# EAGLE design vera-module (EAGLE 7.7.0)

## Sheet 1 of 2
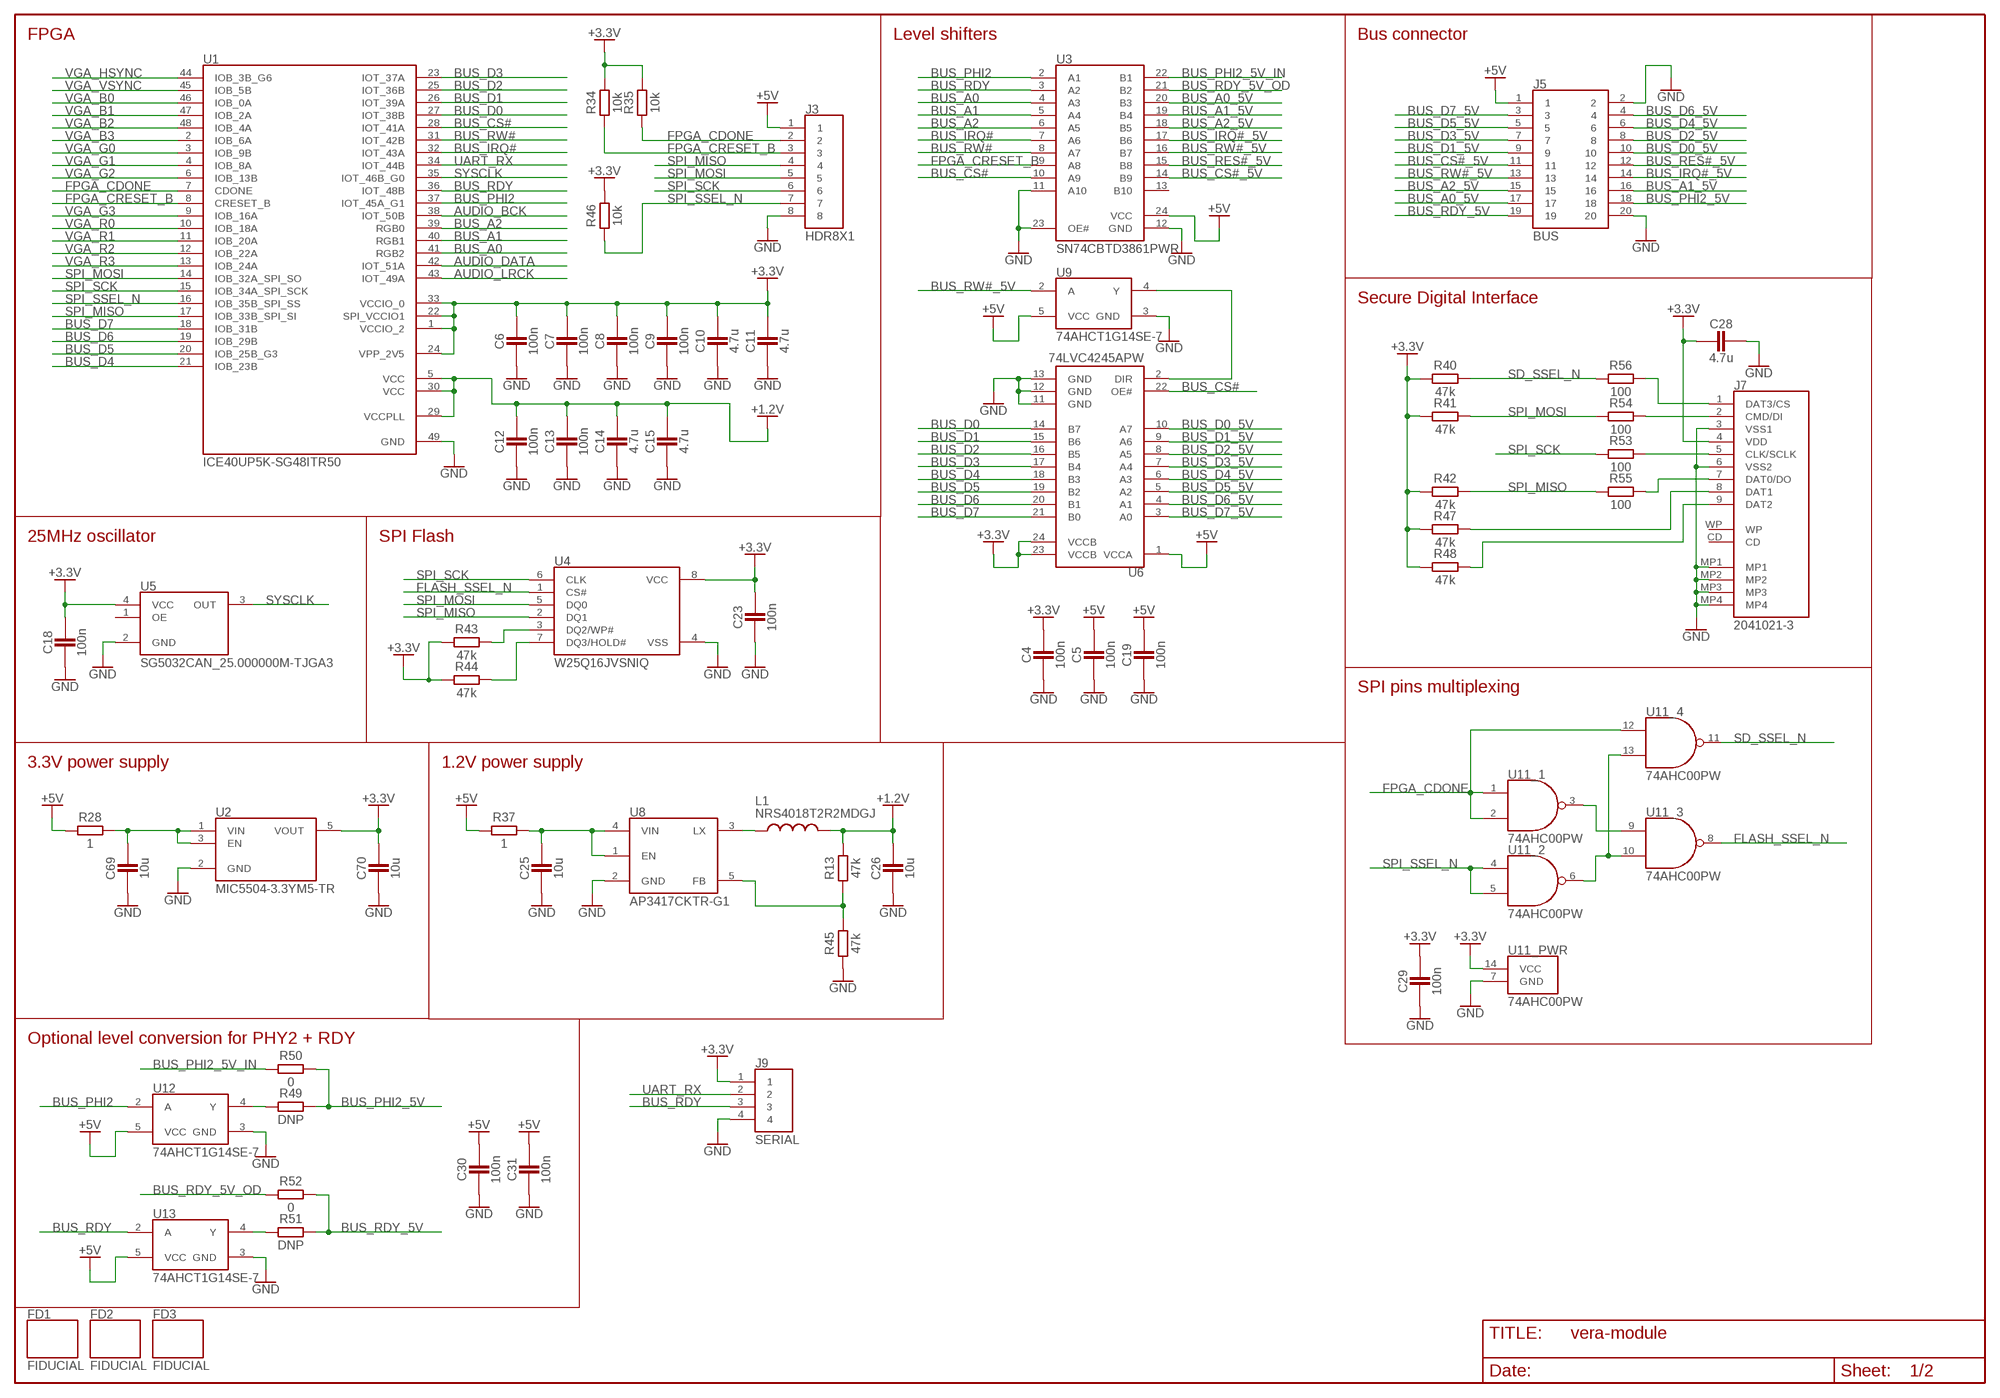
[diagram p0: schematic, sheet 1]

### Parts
C4  100n  CAPACITOR0603  [C0603]
C5  100n  CAPACITOR0603  [C0603]
C6  100n  CAPACITOR0603  [C0603]
C7  100n  CAPACITOR0603  [C0603]
C8  100n  CAPACITOR0603  [C0603]
C9  100n  CAPACITOR0603  [C0603]
C10  4.7u  CAPACITOR0603  [C0603]
C11  4.7u  CAPACITOR0603  [C0603]
C12  100n  CAPACITOR0603  [C0603]
C13  100n  CAPACITOR0603  [C0603]
C14  4.7u  CAPACITOR0603  [C0603]
C15  4.7u  CAPACITOR0603  [C0603]
C18  100n  CAPACITOR0603  [C0603]
C19  100n  CAPACITOR0603  [C0603]
C23  100n  CAPACITOR0603  [C0603]
C25  10u  CAPACITOR0805  [C0805]
C26  10u  CAPACITOR0805  [C0805]
C28  4.7u  CAPACITOR0603  [C0603]
C29  100n  CAPACITOR0603  [C0603]
C30  100n  CAPACITOR0603  [C0603]
C31  100n  CAPACITOR0603  [C0603]
C69  10u  CAPACITOR0805  [C0805]
C70  10u  CAPACITOR0805  [C0805]
FD1  FIDUCIAL  [FIDUCIAL]
FD2  FIDUCIAL  [FIDUCIAL]
FD3  FIDUCIAL  [FIDUCIAL]
J3  HDR8X1  [HDR8X1]
J5  BUS  HDR2X10  [HDR2X10]
J7  2041021-3  [2041021-3]
J9  SERIAL  HDR4X1  [HDR4X1]
L1  NRS4018T2R2MDGJ  INDUCTORNRS4018  [NRS4018]
R13  47k  RESISTOR0603  [R0603]
R28  1  RESISTOR0603  [R0603]
R34  10k  RESISTOR0603  [R0603]
R35  10k  RESISTOR0603  [R0603]
R37  1  RESISTOR0603  [R0603]
R40  47k  RESISTOR0603  [R0603]
R41  47k  RESISTOR0603  [R0603]
R42  47k  RESISTOR0603  [R0603]
R43  47k  RESISTOR0603  [R0603]
R44  47k  RESISTOR0603  [R0603]
R45  47k  RESISTOR0603  [R0603]
R46  10k  RESISTOR0603  [R0603]
R47  47k  RESISTOR0603  [R0603]
R48  47k  RESISTOR0603  [R0603]
R49  DNP  RESISTOR0603  [R0603]
R50  0  RESISTOR0603  [R0603]
R51  DNP  RESISTOR0603  [R0603]
R52  0  RESISTOR0603  [R0603]
R53  100  RESISTOR0603  [R0603]
R54  100  RESISTOR0603  [R0603]
R55  100  RESISTOR0603  [R0603]
R56  100  RESISTOR0603  [R0603]
U1  ICE40UP5K-SG48ITR50  [QFN-48]
U2  MIC5504-3.3YM5-TR  [SOT-23-5]
U3  SN74CBTD3861PWR  [TSSOP-24]
U4  W25Q16JVSNIQ  QSPI_FLASHSOIC8  [SOIC-8]
U5  SG5032CAN_25.000000M-TJGA3  SG5032CAN_40.000000M-TJGA3  [SG5032]
U6  74LVC4245APW  [TSSOP-24]
U8  AP3417CKTR-G1  [SOT-23-5]
U9  74AHCT1G14SE-7  [TSSOP-5]
U11  74AHC00PW  [TSSOP-14]
U12  74AHCT1G14SE-7  [TSSOP-5]
U13  74AHCT1G14SE-7  [TSSOP-5]

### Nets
+1.2V: C12.2 C13.2 C14.2 C15.2 C26.2 L1.2 R13.2 U1.5(VCC) U1.29(VCCPLL) U1.30(VCC)
+3.3V: C4.2 C6.2 C7.2 C8.2 C9.2 C10.2 C11.2 C18.2 C23.2 C28.1 C29.2 C70.2 J7.4(VDD) J9.1 R34.1 R35.1 R40.1 R41.1 R42.1 R43.1 R44.1 R46.1 R47.1 R48.1 U1.1(VCCIO_2) U1.22(SPI_VCCIO1) U1.24(VPP_2V5) U1.33(VCCIO_0) U2.5(VOUT) U4.8(VCC) U5.4(VCC) U6.23(VCCB) U6.24(VCCB) U11.14(_PWR:VCC) ; also sheet 2
+5V [5V]: C5.2 C19.2 C30.2 C31.2 J3.1 J5.1 R28.1 R37.1 U3.24(VCC) U6.1(VCCA) U9.5(VCC) U12.5(VCC) U13.5(VCC)
AUDIO_BCK: U1.38(IOT_50B) ; also sheet 2
AUDIO_DATA: U1.42(IOT_51A) ; also sheet 2
AUDIO_LRCK: U1.43(IOT_49A) ; also sheet 2
BUS_A0: U1.41(RGB2) U3.4(A3)
BUS_A0_5V: J5.17 U3.20(B3)
BUS_A1: U1.40(RGB1) U3.5(A4)
BUS_A1_5V: J5.16 U3.19(B4)
BUS_A2: U1.39(RGB0) U3.6(A5)
BUS_A2_5V: J5.15 U3.18(B5)
BUS_CS#: U1.28(IOT_41A) U3.10(A9) U6.22(OE#)
BUS_CS#_5V: J5.11 U3.14(B9)
BUS_D0: U1.27(IOT_38B) U6.14(B7)
BUS_D0_5V: J5.10 U6.10(A7)
BUS_D1: U1.26(IOT_39A) U6.15(B6)
BUS_D1_5V: J5.9 U6.9(A6)
BUS_D2: U1.25(IOT_36B) U6.16(B5)
BUS_D2_5V: J5.8 U6.8(A5)
BUS_D3: U1.23(IOT_37A) U6.17(B4)
BUS_D3_5V: J5.7 U6.7(A4)
BUS_D4: U1.21(IOB_23B) U6.18(B3)
BUS_D4_5V: J5.6 U6.6(A3)
BUS_D5: U1.20(IOB_25B_G3) U6.19(B2)
BUS_D5_5V: J5.5 U6.5(A2)
BUS_D6: U1.19(IOB_29B) U6.20(B1)
BUS_D6_5V: J5.4 U6.4(A1)
BUS_D7: U1.18(IOB_31B) U6.21(B0)
BUS_D7_5V: J5.3 U6.3(A0)
BUS_IRQ#: U1.32(IOT_43A) U3.7(A6)
BUS_IRQ#_5V: J5.14 U3.17(B6)
BUS_PHI2: U1.37(IOT_45A_G1) U3.2(A1) U12.2(A)
BUS_PHI2_5V: J5.18 R49.2 R50.2
BUS_PHI2_5V_IN: R50.1 U3.22(B1)
BUS_RDY: J9.3 U1.36(IOT_48B) U3.3(A2) U13.2(A)
BUS_RDY_5V: J5.19 R51.2 R52.2
BUS_RDY_5V_OD: R52.1 U3.21(B2)
BUS_RES#_5V: J5.12 U3.15(B8)
BUS_RW#: U1.31(IOT_42B) U3.8(A7)
BUS_RW#_5V: J5.13 U3.16(B7) U9.2(A)
FLASH_SSEL_N: U4.1(CS#) U11.8(_3:Y)
FPGA_CDONE: J3.2 R35.2 U1.7(CDONE) U11.1(_1:A) U11.2(_1:B) U11.12(_4:A)
FPGA_CRESET_B: J3.3 R34.2 U1.8(CRESET_B) U3.9(A8)
GND: C4.1 C5.1 C6.1 C7.1 C8.1 C9.1 C10.1 C11.1 C12.1 C13.1 C14.1 C15.1 C18.1 C19.1 C23.1 C25.1 C26.1 C28.2 C29.1 C30.1 C31.1 C69.1 C70.1 J3.8 J5.2 J5.20 J7.3(VSS1) J7.6(VSS2) J7.MP1 J7.MP2 J7.MP3 J7.MP4 J9.4 R45.1 U1.49(GND) U2.2(GND) U3.11(A10) U3.12(GND) U3.23(OE#) U4.4(VSS) U5.2(GND) U6.11(GND) U6.12(GND) U6.13(GND) U8.2(GND) U9.3(GND) U11.7(_PWR:GND) U12.3(GND) U13.3(GND) ; also sheet 2
N$7: C69.2 R28.2 U2.1(VIN) U2.3(EN)
N$8: U6.2(DIR) U9.4(Y)
N$14: R43.2 U4.3(DQ2/WP#)
N$15: R13.1 R45.2 U8.5(FB)
N$19: R44.2 U4.7(DQ3/HOLD#)
N$20: L1.1 U8.3(LX)
N$22 [5V]: C25.2 R37.2 U8.1(EN) U8.4(VIN)
N$43: J7.8(DAT1) R47.2
N$44: J7.9(DAT2) R48.2
N$46: U11.3(_1:Y) U11.9(_3:A)
N$47: U11.6(_2:Y) U11.10(_3:B) U11.13(_4:B)
N$48: R49.1 U12.4(Y)
N$50: R51.1 U13.4(Y)
N$51: J7.2(CMD/DI) R54.2
N$52: J7.5(CLK/SCLK) R53.2
N$53: J7.1(DAT3/CS) R56.2
N$54: J7.7(DAT0/DO) R55.2
SD_SSEL_N: R40.2 R56.1 U11.11(_4:Y)
SPI_MISO: J3.4 R42.2 R55.1 U1.17(IOB_33B_SPI_SI) U4.2(DQ1)
SPI_MOSI: J3.5 R41.2 R54.1 U1.14(IOB_32A_SPI_SO) U4.5(DQ0)
SPI_SCK: J3.6 R53.1 U1.15(IOB_34A_SPI_SCK) U4.6(CLK)
SPI_SSEL_N: J3.7 R46.2 U1.16(IOB_35B_SPI_SS) U11.4(_2:A) U11.5(_2:B)
SYSCLK: U1.35(IOT_46B_G0) U5.3(OUT) ; also sheet 2
UART_RX: J9.2 U1.34(IOT_44B)
VGA_B0: U1.46(IOB_0A) ; also sheet 2
VGA_B1: U1.47(IOB_2A) ; also sheet 2
VGA_B2: U1.48(IOB_4A) ; also sheet 2
VGA_B3: U1.2(IOB_6A) ; also sheet 2
VGA_G0: U1.3(IOB_9B) ; also sheet 2
VGA_G1: U1.4(IOB_8A) ; also sheet 2
VGA_G2: U1.6(IOB_13B) ; also sheet 2
VGA_G3: U1.9(IOB_16A) ; also sheet 2
VGA_HSYNC: U1.44(IOB_3B_G6) ; also sheet 2
VGA_R0: U1.10(IOB_18A) ; also sheet 2
VGA_R1: U1.11(IOB_20A) ; also sheet 2
VGA_R2: U1.12(IOB_22A) ; also sheet 2
VGA_R3: U1.13(IOB_24A) ; also sheet 2
VGA_VSYNC: U1.45(IOB_5B) ; also sheet 2
Unconnected: J7.CD J7.WP U3.13(B10) U5.1(OE)

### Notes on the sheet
- FPGA | Level shifters | Bus connector
- Secure Digital Interface
- 25MHz oscillator | SPI Flash
- SPI pins multiplexing
- 3.3V power supply | 1.2V power supply
- Optional level conversion for PHY2 + RDY

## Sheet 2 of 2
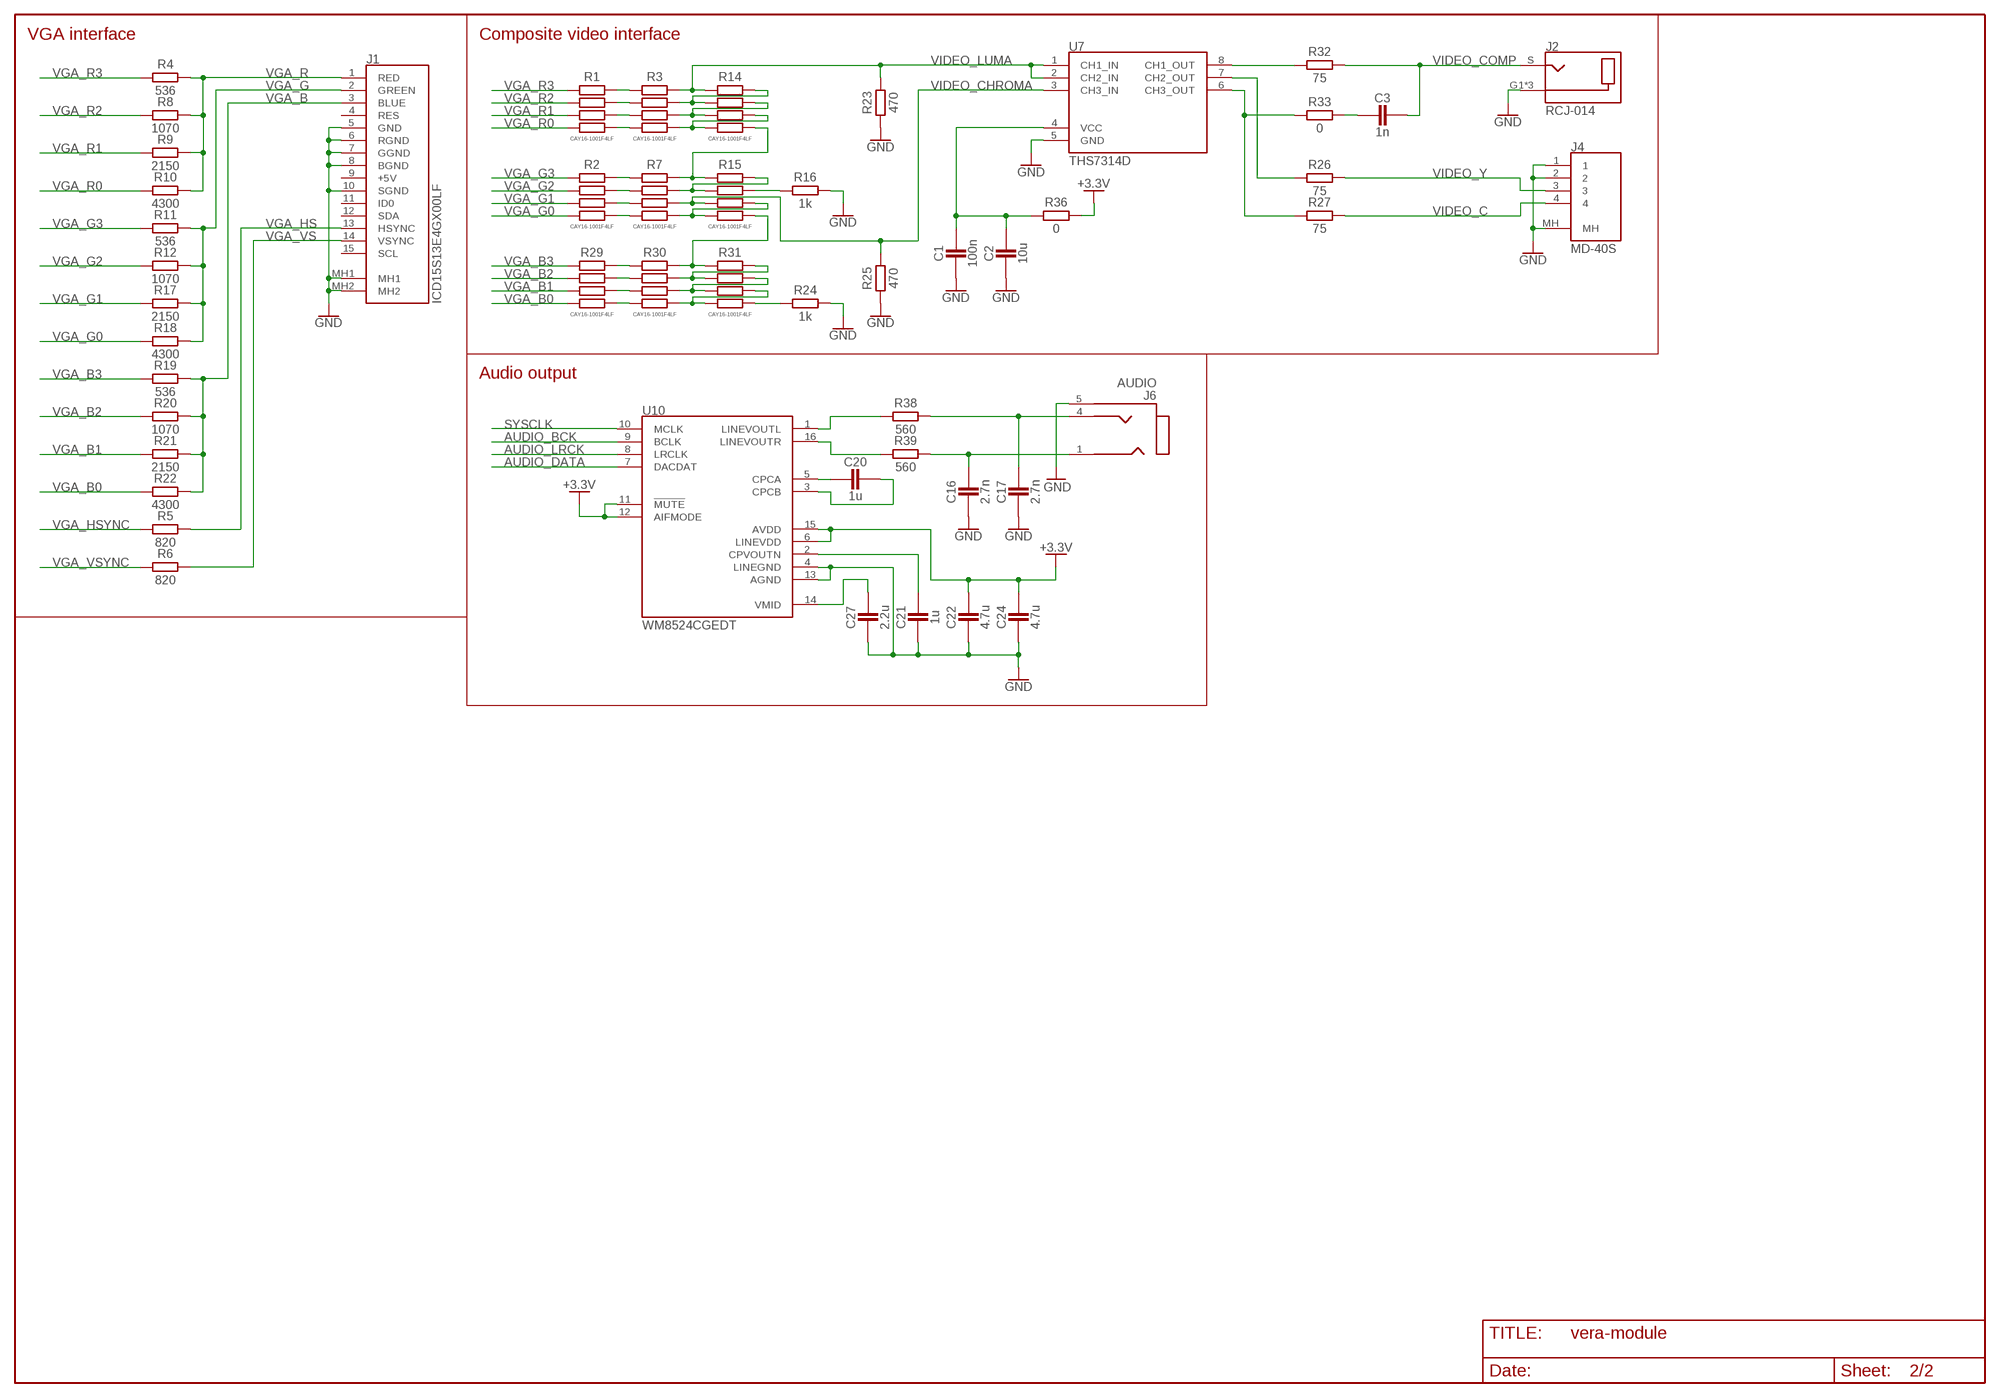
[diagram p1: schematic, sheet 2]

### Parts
C1  100n  CAPACITOR0603  [C0603]
C2  10u  CAPACITOR0805  [C0805]
C3  1n  CAPACITOR0603  [C0603]
C16  2.7n  CAPACITOR0603  [C0603]
C17  2.7n  CAPACITOR0603  [C0603]
C20  1u  CAPACITOR0603  [C0603]
C21  1u  CAPACITOR0603  [C0603]
C22  4.7u  CAPACITOR0603  [C0603]
C24  4.7u  CAPACITOR0603  [C0603]
C27  2.2u  CAPACITOR0603  [C0603]
J1  ICD15S13E4GX00LF  [1-1734344-2]
J2  RCJ-014  [RCJ-01X]
J4  MD-40S  [MD-40S]
J6  AUDIO  35RASMT2BHNTRX  [35RASMT2BHNTRX]
R1  CAY16-1001F4LF  RES_ARRAY41206  [RA4_1206]
R2  CAY16-1001F4LF  RES_ARRAY41206  [RA4_1206]
R3  CAY16-1001F4LF  RES_ARRAY41206  [RA4_1206]
R4  536  RESISTOR0603  [R0603]
R5  820  RESISTOR0603  [R0603]
R6  820  RESISTOR0603  [R0603]
R7  CAY16-1001F4LF  RES_ARRAY41206  [RA4_1206]
R8  1070  RESISTOR0603  [R0603]
R9  2150  RESISTOR0603  [R0603]
R10  4300  RESISTOR0603  [R0603]
R11  536  RESISTOR0603  [R0603]
R12  1070  RESISTOR0603  [R0603]
R14  CAY16-1001F4LF  RES_ARRAY41206  [RA4_1206]
R15  CAY16-1001F4LF  RES_ARRAY41206  [RA4_1206]
R16  1k  RESISTOR0603  [R0603]
R17  2150  RESISTOR0603  [R0603]
R18  4300  RESISTOR0603  [R0603]
R19  536  RESISTOR0603  [R0603]
R20  1070  RESISTOR0603  [R0603]
R21  2150  RESISTOR0603  [R0603]
R22  4300  RESISTOR0603  [R0603]
R23  470  RESISTOR0603  [R0603]
R24  1k  RESISTOR0603  [R0603]
R25  470  RESISTOR0603  [R0603]
R26  75  RESISTOR0603  [R0603]
R27  75  RESISTOR0603  [R0603]
R29  CAY16-1001F4LF  RES_ARRAY41206  [RA4_1206]
R30  CAY16-1001F4LF  RES_ARRAY41206  [RA4_1206]
R31  CAY16-1001F4LF  RES_ARRAY41206  [RA4_1206]
R32  75  RESISTOR0603  [R0603]
R33  0  RESISTOR0603  [R0603]
R36  0  RESISTOR0603  [R0603]
R38  560  RESISTOR0603  [R0603]
R39  560  RESISTOR0603  [R0603]
U7  THS7314D  [SOIC-8]
U10  WM8524CGEDT  [TSSOP-16]

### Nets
+3.3V: C22.2 C24.2 R36.2 U10.6(LINEVDD) U10.11(!MUTE) U10.12(AIFMODE) U10.15(AVDD) ; also sheet 1
AUDIO_BCK: U10.9(BCLK) ; also sheet 1
AUDIO_DATA: U10.7(DACDAT) ; also sheet 1
AUDIO_LRCK: U10.8(LRCLK) ; also sheet 1
GND: C1.1 C2.1 C16.1 C17.1 C21.1 C22.1 C24.1 C27.1 J1.5(GND) J1.6(RGND) J1.7(GGND) J1.8(BGND) J1.10(SGND) J1.MH1 J1.MH2 J2.G1(G) J2.G2(G) J2.G3(G) J4.1 J4.2 J4.MH J6.5(SLEEVE) R16.2 R23.1 R24.2 R25.1 U7.5(GND) U10.4(LINEGND) U10.13(AGND) ; also sheet 1
N$1: R1.1A R3.1B
N$2: R1.2A R3.2B
N$3: R1.3A R3.3B
N$4: R1.4A R3.4B
N$5: R2.1A R7.1B
N$6: R2.2A R7.2B
N$9: R29.1A R30.1B
N$10: R2.3A R7.3B
N$11: R2.4A R7.4B
N$12: R27.1 R33.1 U7.6(CH3_OUT)
N$13: R3.2A R14.1A R14.2B
N$16: R3.3A R14.2A R14.3B
N$17: R3.4A R14.3A R14.4B
N$18: R7.1A R14.4A R15.1B
N$21: R7.2A R15.1A R15.2B
N$23: R32.1 U7.8(CH1_OUT)
N$24: C3.1 R33.2
N$25: R7.4A R15.3A R15.4B
N$26: C20.2 U10.3(CPCB)
N$27: R29.2A R30.2B
N$28: R29.3A R30.3B
N$29: R15.2A R16.1
N$30: R29.4A R30.4B
N$31: R15.4A R30.1A R31.1B
N$32: R30.2A R31.1A R31.2B
N$33: R30.3A R31.2A R31.3B
N$34: R24.1 R31.4A
N$35: R30.4A R31.3A R31.4B
N$36: R26.1 U7.7(CH2_OUT)
N$37: C1.2 C2.2 R36.1 U7.4(VCC)
N$38: C17.2 J6.4(TIP) R38.2
N$39: C16.2 J6.1(RING) R39.2
N$40: R38.1 U10.1(LINEVOUTL)
N$41: R39.1 U10.16(LINEVOUTR)
N$42: C20.1 U10.5(CPCA)
N$45: C21.2 U10.2(CPVOUTN)
N$49: C27.2 U10.14(VMID)
SYSCLK: U10.10(MCLK) ; also sheet 1
VGA_B: J1.3(BLUE) R19.2 R20.2 R21.2 R22.2
VGA_B0: R22.1 R29.4B ; also sheet 1
VGA_B1: R21.1 R29.3B ; also sheet 1
VGA_B2: R20.1 R29.2B ; also sheet 1
VGA_B3: R19.1 R29.1B ; also sheet 1
VGA_G: J1.2(GREEN) R11.2 R12.2 R17.2 R18.2
VGA_G0: R2.4B R18.1 ; also sheet 1
VGA_G1: R2.3B R17.1 ; also sheet 1
VGA_G2: R2.2B R12.1 ; also sheet 1
VGA_G3: R2.1B R11.1 ; also sheet 1
VGA_HS: J1.13(HSYNC) R5.2
VGA_HSYNC: R5.1 ; also sheet 1
VGA_R: J1.1(RED) R4.2 R8.2 R9.2 R10.2
VGA_R0: R1.4B R10.1 ; also sheet 1
VGA_R1: R1.3B R9.1 ; also sheet 1
VGA_R2: R1.2B R8.1 ; also sheet 1
VGA_R3: R1.1B R4.1 ; also sheet 1
VGA_VS: J1.14(VSYNC) R6.2
VGA_VSYNC: R6.1 ; also sheet 1
VIDEO_C: J4.4 R27.2
VIDEO_CHROMA: R7.3A R15.3B R25.2 U7.3(CH3_IN)
VIDEO_COMP: C3.2 J2.S R32.2
VIDEO_LUMA: R3.1A R14.1B R23.2 U7.1(CH1_IN) U7.2(CH2_IN)
VIDEO_Y: J4.3 R26.2
Unconnected: J1.4(RES) J1.9(+5V) J1.11(ID0) J1.12(SDA) J1.15(SCL)

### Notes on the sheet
- VGA interface | Composite video interface
- Audio output

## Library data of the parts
C1-C31 C69 C70 = rcl:CAPACITOR
FD1-FD3 = misc:FIDUCIAL
J1 = connectors:ICD15S13E4GX00LF
J2 = connectors:RCJ-014
J3 = connectors:HDR8X1
J4 = connectors:MD-40S
J5 = connectors:HDR2X10
J6 = connectors:35RASMT2BHNTRX
J7 = connectors:2041021-3
J9 = connectors:HDR4X1
L1 = rcl:INDUCTOR
R1-R3 R7 R14 R15 R29-R31 = rcl:RES_ARRAY4
R4-R6 R8-R13 R16-R28 R32-R56 = rcl:RESISTOR
U1 = integrated_circuits:ICE40UP5K-SG48ITR50: Lattice ICE40 5K LE FPGA
U2 = integrated_circuits:MIC5504-3.3YM5-TR
U3 = integrated_circuits:SN74CBTD3861PWR
U4 = integrated_circuits:QSPI_FLASH
U5 = integrated_circuits:SG5032CAN_40.000000M-TJGA3: Epson 40 MHz 3.3V Oscillator +/- 50ppm
U6 = integrated_circuits:74LVC4245APW
U7 = integrated_circuits:THS7314D
U8 = integrated_circuits:AP3417CKTR-G1
U9 U12 U13 = integrated_circuits:74AHCT1G14SE-7
U10 = integrated_circuits:WM8524CGEDT
U11 = integrated_circuits:74AHC00PW

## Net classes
1 5V: clearance 0.2 mm

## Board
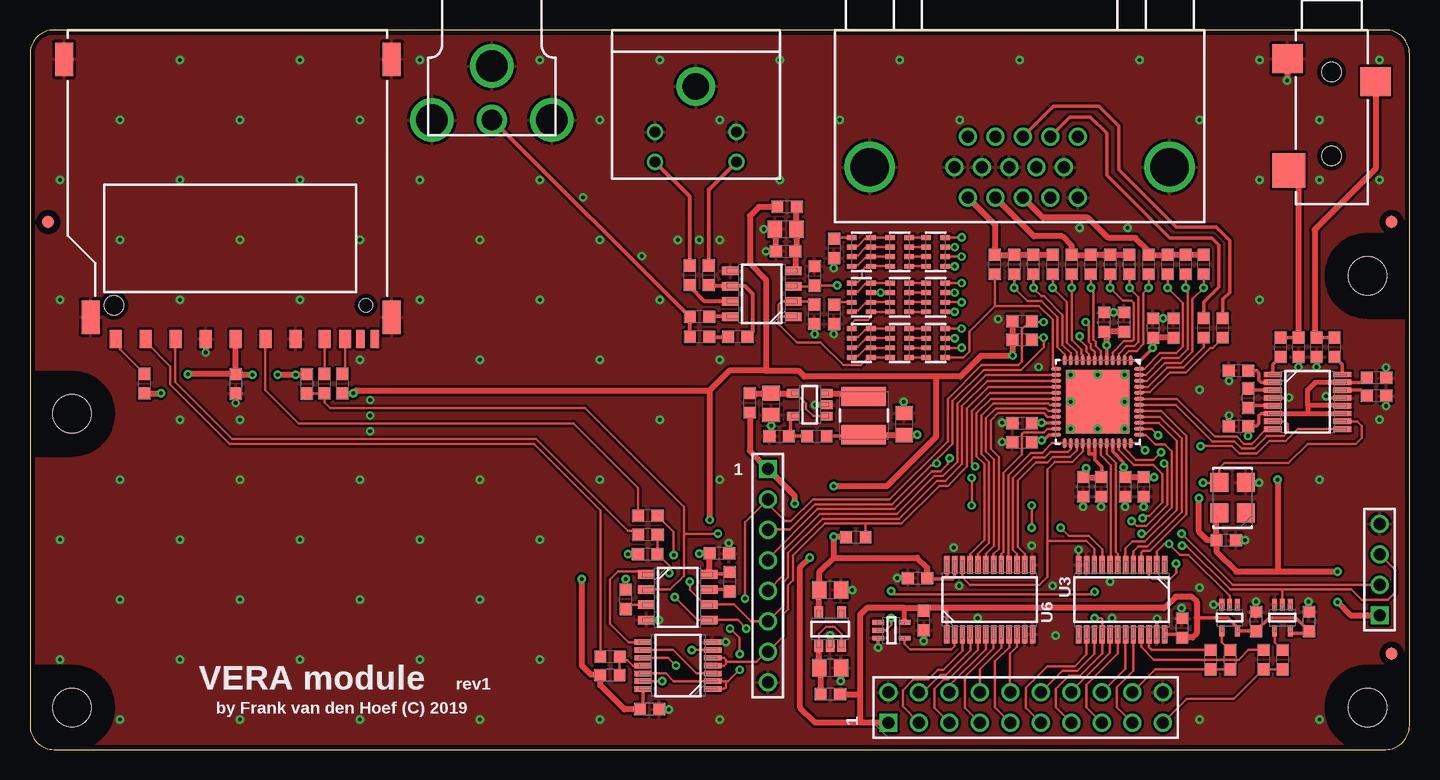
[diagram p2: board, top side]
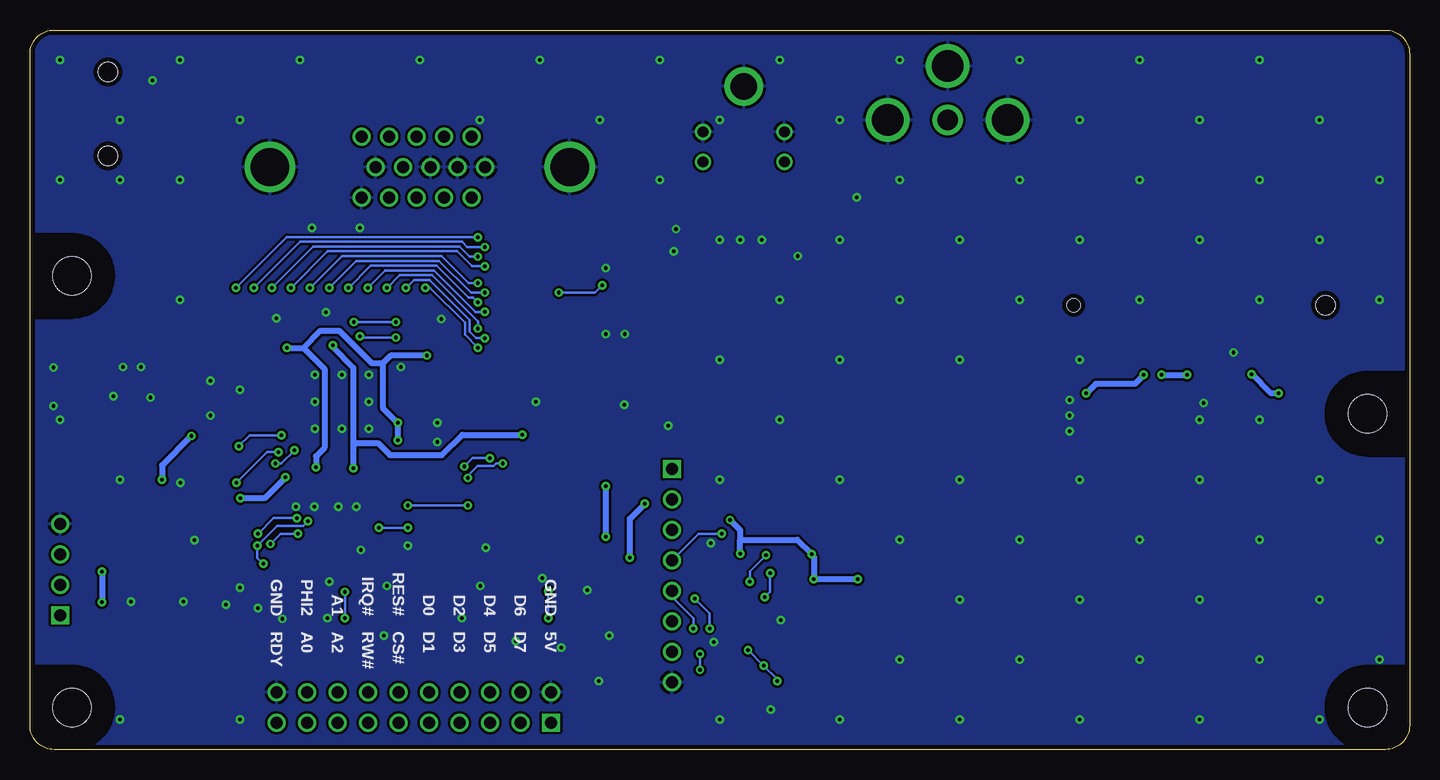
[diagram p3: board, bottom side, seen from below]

Size 115 x 60 mm. Coordinates in mm from the lower left corner, seen from the top.
Outline: 115,2 115,58 arc90 113,60 2,60 arc90 0,58 0,2 arc90 2,0 113,0 arc90 115,2
Copper layers (1*16): Top 0.035mm / dielectric 1.6mm / Bottom 0.035mm
Design rules "Frank_2-layer *": minimum track width 0.2mm, minimum drill 0.3mm, track to track 0.2mm, track to pad 0.2mm, pad to pad 0.2mm, via to via 0.2mm, smd to smd 0mil, copper to edge 0.4mm, drill to drill 10mil, minimum pad ring 0.2mm, minimum via ring 0.2mm, stop-mask expansion 0.1mm, vias tented up to drill 20mil, thermal gap 10mil
Holes 3.2 mm at 3.5,28 3.5,3.5 111.5,3.5 111.5,39.5
tRestrict: area 86,26 to 92,32; area 0,24.5 to 7,31.5; area 0,0 to 7,7; area 108,0 to 115,7; area 108,36 to 115,43
bRestrict: area 0,24.5 to 7,31.5; area 0,0 to 7,7; area 108,0 to 115,7; area 108,36 to 115,43

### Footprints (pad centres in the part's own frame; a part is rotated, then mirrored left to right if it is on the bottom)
C0603 = smd 0.95 x 1: 1 -0.8,0; 2 0.8,0
C0805 = smd 1.15 x 1.45: 1 -0.9,0; 2 0.9,0
FIDUCIAL = smd 1 x 1: FD 0,0
1-1734344-2 = drill 1: 1 4.315,13.97; 2 2.025,13.97; 3 -0.265,13.97; 4 -2.555,13.97; 5 -4.845,13.97; 6 5.455,11.43; 7 3.165,11.43; 8 0.875,11.43; 9 -1.415,11.43; 10 -3.705,11.43; 11 4.315,8.89; 12 2.025,8.89; 13 -0.265,8.89; 14 -2.555,8.89; 15 -4.845,8.89 | drill 3.18: MH1 -12.495,11.43; MH2 12.495,11.43
RCJ-01X = drill 2.6: G1 0,0; G2 -5,-4.5; G3 5,-4.5 | drill 1.7: S 0,-4.5
HDR8X1 = drill 1 square: 1 0,8.89 | drill 1: 2 0,6.35; 3 0,3.81; 4 0,1.27; 5 0,-1.27; 6 0,-3.81; 7 0,-6.35; 8 0,-8.89
MD-40S = drill 0.9: 1 -3.4,-8.5; 2 3.4,-8.5; 3 -3.4,-11; 4 3.4,-11 | drill 2.2: MH 0,-4.7
HDR2X10 = drill 1 square: 1 -1.27,11.43 | drill 1: 2 1.27,11.43; 3 -1.27,8.89; 4 1.27,8.89; 5 -1.27,6.35; 6 1.27,6.35; 7 -1.27,3.81; 8 1.27,3.81; 9 -1.27,1.27; 10 1.27,1.27; 11 -1.27,-1.27; 12 1.27,-1.27; 13 -1.27,-3.81; 14 1.27,-3.81; 15 -1.27,-6.35; 16 1.27,-6.35; 17 -1.27,-8.89; 18 1.27,-8.89; 19 -1.27,-11.43; 20 1.27,-11.43
35RASMT2BHNTRX = smd 2.4 x 2.55: 1 4.3,3.675; 5 2.4,-3.675 | smd 2.9 x 2.75: 4 11.7,-3.575 | hole 1.6: 3.5,0; 10.5,0
2041021-3 = smd 1 x 1.5: 1 6.875,25.75; 2 4.375,25.75; 3 1.875,25.75; 4 -0.625,25.75; 5 -3.125,25.75; 6 -5.625,25.75; 7 -8.055,25.75; 8 -9.755,25.75; 9 9.375,25.75 | smd 0.7 x 1.5: CD -11.055,25.75; WP -12.255,25.75 | smd 1.5 x 2.8: MP1 -13.65,23.95; MP2 11.45,23.95; MP3 -13.65,2.45; MP4 13.65,2.45 | hole 1.1: -11.5,22.95 | hole 1.6: 9.5,22.95
HDR4X1 = drill 1 square: 1 0,3.81 | drill 1: 2 0,1.27; 3 0,-1.27; 4 0,-3.81
NRS4018 = smd 1.6 x 3.7: 1 -1.6,0; 2 1.6,0
RA4_1206 = smd 0.4 x 0.8: 1A -1.2,0.8; 1B -1.2,-0.8; 2A -0.4,0.8; 2B -0.4,-0.8; 3A 0.4,0.8; 3B 0.4,-0.8; 4A 1.2,0.8; 4B 1.2,-0.8
R0603 = smd 0.95 x 1: 1 -0.8,0; 2 0.8,0
QFN-48 = smd 0.85 x 0.3: 1 -3.45,2.75; 2 -3.45,2.25; 3 -3.45,1.75; 4 -3.45,1.25; 5 -3.45,0.75; 6 -3.45,0.25; 7 -3.45,-0.25; 8 -3.45,-0.75; 9 -3.45,-1.25; 10 -3.45,-1.75; 11 -3.45,-2.25; 12 -3.45,-2.75; 25 3.45,-2.75; 26 3.45,-2.25; 27 3.45,-1.75; 28 3.45,-1.25; 29 3.45,-0.75; 30 3.45,-0.25; 31 3.45,0.25; 32 3.45,0.75; 33 3.45,1.25; 34 3.45,1.75; 35 3.45,2.25; 36 3.45,2.75 | smd 0.3 x 0.85: 13 -2.75,-3.45; 14 -2.25,-3.45; 15 -1.75,-3.45; 16 -1.25,-3.45; 17 -0.75,-3.45; 18 -0.25,-3.45; 19 0.25,-3.45; 20 0.75,-3.45; 21 1.25,-3.45; 22 1.75,-3.45; 23 2.25,-3.45; 24 2.75,-3.45; 37 2.75,3.45; 38 2.25,3.45; 39 1.75,3.45; 40 1.25,3.45; 41 0.75,3.45; 42 0.25,3.45; 43 -0.25,3.45; 44 -0.75,3.45; 45 -1.25,3.45; 46 -1.75,3.45; 47 -2.25,3.45; 48 -2.75,3.45 | smd 5.3 x 5.3: 49 0,0
SOT-23-5 = smd 1 x 0.71: 1 -1.4,0.95; 2 -1.4,0; 3 -1.4,-0.95; 4 1.4,-0.95; 5 1.4,0.95
TSSOP-24 = smd 1.5 x 0.45: 1 -2.9,3.575; 2 -2.9,2.925; 3 -2.9,2.275; 4 -2.9,1.625; 5 -2.9,0.975; 6 -2.9,0.325; 7 -2.9,-0.325; 8 -2.9,-0.975; 9 -2.9,-1.625; 10 -2.9,-2.275; 11 -2.9,-2.925; 12 -2.9,-3.575; 13 2.9,-3.575; 14 2.9,-2.925; 15 2.9,-2.275; 16 2.9,-1.625; 17 2.9,-0.975; 18 2.9,-0.325; 19 2.9,0.325; 20 2.9,0.975; 21 2.9,1.625; 22 2.9,2.275; 23 2.9,2.925; 24 2.9,3.575
SOIC-8 = smd 1.35 x 0.71: 1 -2.625,1.905; 2 -2.625,0.635; 3 -2.625,-0.635; 4 -2.625,-1.905; 5 2.625,-1.905; 6 2.625,-0.635; 7 2.625,0.635; 8 2.625,1.905
SG5032 = smd 1.6 x 1.5: 1 -1.27,-1.1; 2 1.27,-1.1; 3 1.27,1.1; 4 -1.27,1.1
TSSOP-5 = smd 0.95 x 0.4: 1 -1.1,0.65; 2 -1.1,0; 3 -1.1,-0.65; 4 1.1,-0.65; 5 1.1,0.65
TSSOP-16 = smd 1.5 x 0.45: 1 -2.9,2.275; 2 -2.9,1.625; 3 -2.9,0.975; 4 -2.9,0.325; 5 -2.9,-0.325; 6 -2.9,-0.975; 7 -2.9,-1.625; 8 -2.9,-2.275; 9 2.9,-2.275; 10 2.9,-1.625; 11 2.9,-0.975; 12 2.9,-0.325; 13 2.9,0.325; 14 2.9,0.975; 15 2.9,1.625; 16 2.9,2.275
TSSOP-14 = smd 1.45 x 0.45: 1 -2.9,1.95; 2 -2.9,1.3; 3 -2.9,0.65; 4 -2.9,0; 5 -2.9,-0.65; 6 -2.9,-1.3; 7 -2.9,-1.95; 8 2.9,-1.95; 9 2.9,-1.3; 10 2.9,-0.65; 11 2.9,0; 12 2.9,0.65; 13 2.9,1.3; 14 2.9,1.95

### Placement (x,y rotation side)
C1  63,41.55 0 top
C2  63,43.4 0 top
C3  55.8,34.4 180 top
C4  74,14.3 0 top
C5  96,10.15 270 top
C6  93.6,35.15 270 top
C7  82.7,27.25 0 top
C8  82.7,25.65 0 top
C9  91.3,21.9 90 top
C10  92.85,21.9 90 top
C11  95.3,35.15 270 top
C12  89.5,35.65 270 top
C13  89.3,21.9 90 top
C14  87.8,21.9 90 top
C15  91.2,35.65 270 top
C16  107.25,33.55 90 top
C17  105.75,33.55 90 top
C18  99.7,17.45 180 top
C19  74.5,10.75 90 top
C20  101.55,29.3 90 top
C21  100.75,31.6 0 top
C22  100.75,27 0 top
C23  57.45,16.35 180 top
C24  112.25,31 180 top
C25  61.8,28.8 90 top
C26  72.85,27.15 270 top
C27  112.25,29.5 180 top
C28  17.15,30.5 270 top
C29  51.65,3.35 180 top
C30  102.2,10.7 270 top
C31  106.6,10.7 270 top
C69  66.7,6.8 180 top
C70  66.7,13.3 180 top
FD1  1.5,44 0 top
FD2  113.5,8 0 top
FD3  113.5,44 0 top
J1  82.5,60 180 top
J2  38.5,57 0 top
J3  61.5,14.5 0 top
J4  55.5,60 0 top
J5  83,3.5 90 top
J6  108.5,60 270 top
J7  16.5,60 180 top
J9  112.5,15 180 top
L1  69.5,27.85 270 top
R1  75.5,33.9 90 top
R2  75.5,37.7 90 top
R3  72.5,33.9 90 top
R4  80.45,40.45 90 top
R5  99.45,35.15 90 top
R6  97.85,35.15 90 top
R7  72.5,37.7 90 top
R8  82.05,40.45 90 top
R9  83.65,40.45 90 top
R10  85.25,40.45 90 top
R11  86.85,40.45 90 top
R12  88.45,40.45 90 top
R13  65.6,26.15 0 top
R14  69.3,33.9 90 top
R15  69.3,37.7 90 top
R16  67,36.3 270 top
R17  90.05,40.45 90 top
R18  91.65,40.45 90 top
R19  93.25,40.45 90 top
R20  94.85,40.45 90 top
R21  96.35,40.45 90 top
R22  97.85,40.45 90 top
R23  65.4,36.3 90 top
R24  67,41.8 270 top
R25  65.4,39.5 270 top
R26  55,39.55 90 top
R27  56.6,39.55 90 top
R28  66.7,4.6 180 top
R29  75.5,41.5 90 top
R30  72.5,41.5 90 top
R31  69.3,41.5 90 top
R32  55.8,36.05 180 top
R33  59,34.4 180 top
R34  82.7,34.2 0 top
R35  82.7,35.75 0 top
R36  63.1,45.25 180 top
R37  60,28.9 90 top
R38  104.25,33.55 90 top
R39  108.75,33.55 90 top
R40  48.35,6.25 0 top
R41  51.5,16.3 0 top
R42  23.05,30.5 270 top
R43  49.65,12.55 270 top
R44  58.3,14 270 top
R45  62.45,26.15 0 top
R46  68.85,17.75 0 top
R47  26.05,30.5 90 top
R48  9.55,30.5 90 top
R49  100,7.5 270 top
R50  98.4,7.5 270 top
R51  104.4,7.5 270 top
R52  102.8,7.5 270 top
R53  51.5,19.5 180 top
R54  51.5,17.9 180 top
R55  24.55,30.5 90 top
R56  48.35,7.75 180 top
U1  89,29 270 top
U2  66.7,10.05 90 top
U3  91,12.5 270 top
U4  54,12.7 0 top
U5  100.25,21 90 top
U6  80,12.5 90 top
U7  61,38 180 top
U8  65,28.75 180 top
U9  71.8,9.95 0 top
U10  106.5,29 0 top
U11  54,7 180 top
U12  100,11 270 top
U13  104.4,11 270 top

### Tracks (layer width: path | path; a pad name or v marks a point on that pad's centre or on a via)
+1.2V  (via drill 0.3)
  Top 0.3: U1.5 v89.75,33.7 | U1.30 88.75,24.65 | 88.75,24.65 88.75,24.15 89.35,23.55 89.35,22.75 | R13.2 67.95,26.15 | U1.29 88.25,24.65 88.75,24.65
  Top 0.5: v89.75,33.7 89.75,34.6 C12.2 C15.2 | 89.35,22.75 C13.2 C14.2 88.05,22.95 v88.05,23.45 | 67.95,26.15 68.05,26.25 L1.2 C26.2 v73.95,26.25
  Bottom 0.5: v89.75,33.7 89.75,33.55 88.05,31.85 88.05,25.55 | 88.05,25.55 v88.05,23.45 | 88.05,25.55 86,25.55 85,24.55 80.65,24.55 78.95,26.25 v73.95,26.25
+3.3V  (via drill 0.3)
  Top 0.3: U1.22 v84.35,27.25 | U1.24 84.95,26.25 84.5,25.8 v84.35,25.8 | U1.33 90.25,24.85 91.15,23.95 v91.15,23.55 | U1.1 92.55,32.45 v93.6,33.5 | 56.65,14.63 58.13,14.63 R44.1 | U6.23 77.08,14.38 76.95,14.25 76.35,14.25 | U6.24 76.42,14.32 76.35,14.25 | 76.35,14.25 74.85,14.25 C4.2 | U10.6 102.62,28.02 102.45,27.85 102.45,27.2 102.25,27 C22.2 | U10.15 111.08,30.62 C24.2 | C29.2 51.1,3.6 U11.14
  Top 0.4: U10.15 107.12,30.62 106.5,30 106.5,28.7 | U10.6 106.5,28.02 | 106.5,28.02 U10.11 | U10.12 106.53,28.68 106.5,28.7 | 106.5,28.7 106.5,28.02
  Top 0.5: C7.2 v84.35,27.25 | C8.2 83.65,25.8 v84.35,25.8 | v91.15,23.55 91.15,22.85 C9.2 C10.2 v93.7,22.7 | C11.2 C6.2 v93.6,33.5 | U4.8 56.65,14.63 C23.2 v55.8,16.35 | 99.13,19.75 U5.4 98.9,19.48 C18.2 | R35.1 R34.1 v81.9,32.85 79.3,32.85 77.55,31.1 75.5,31.1 | U2.5 65.75,13.25 C70.2 65.8,14.8 67,16 | C18.2 98.15,17.45 97.45,18.15 v97.45,20.95 | C22.2 v101.55,26.15 | C28.1 17.15,34.23 J7.4 | C28.1 v13.15,31.3 | R48.1 v10.9,29.7 | R47.1 v26.95,29.7 27.2,29.95 56.65,29.95 | R42.1 23,31.25 v22.15,31.25 v20.65,31.25 | v18.55,31.25 17.2,31.25 C28.1 | R41.1 v49.85,16.3 | R43.1 v49.65,14.2 | C29.2 49.55,3.35 47.55,5.35 R40.1 46.75,6.25 46,7 v46,14.2 | 67,16 73.95,16 74.8,15.15 C4.2 | 67,16 v67,17.75 R46.1 | 75.5,31.1 64.55,31.1 64.05,31.6 61.35,31.6 | 75.5,31.1 75.5,26.05 71.4,21.95 v67,21.95 | R36.2 60.75,45.25 60,44.5 60,40.55 61.35,39.2 61.35,31.6 | 61.35,31.6 58.3,31.6 56.65,29.95 | 56.65,29.95 v56.65,19.15 | C18.2 98.9,16.5 100.55,14.85 104,14.85 | 104,14.85 v109,14.85 | v109,12.3 110.1,11.2 111.5,11.2 111.51,11.19 J9.1 | v104,22.5 104,14.85
  Bottom 0.5: v84.35,25.8 v84.35,27.25 85.6,28.5 85.6,32.2 | v93.6,33.5 92.2,33.5 | 92.2,33.5 90.45,31.75 90.45,25.15 91.15,24.45 v91.15,23.55 | v81.9,32.85 84.95,32.85 85.6,32.2 | 85.6,32.2 86.5,32.2 89.2,34.9 90.8,34.9 92.2,33.5 | v93.7,22.7 95.45,20.95 v97.45,20.95 | v10.9,29.7 11.55,29.7 v13.15,31.3 | v22.15,31.25 22.9,30.5 26.15,30.5 v26.95,29.7 | v20.65,31.25 v18.55,31.25 | v56.65,19.15 55.8,18.3 55.8,17.5 | v55.8,16.35 55.8,17.5 | 55.8,17.5 51.05,17.5 v49.85,16.3 49.65,16.1 v49.65,14.2 v46,14.2 | v67,17.75 v67,21.95 | v109,14.85 v109,12.3 | v101.55,26.15 104,23.7 v104,22.5
+5V  (via drill 0.3)
  Top 0.3: U3.24 95.75,9.6 C5.2 | U6.1 76.42,11.68 76.55,11.8 | U13.5 105.05,9.7 106.4,9.7 C31.2 105.5,11 103.3,11 C30.2 U12.5 100.65,10.2 99.85,11 97.25,11
  Top 0.4: U9.5 72.9,11.8
  Top 0.5: C5.2 96.9,9.35 97.25,9.7 97.25,11 97.25,12.35 96.85,12.75 95.5,12.75 94.55,11.8 76.55,11.8 74.75,11.8 C19.2 74.25,11.8 72.9,11.8 69.75,11.8 69.2,11.25 69.2,4.6 | R37.1 60,24.9 61.45,23.45 61.45,23.44 J3.1 63.75,21.14 v63.75,20.5 | R28.1 69.2,4.6 | J5.1 69.2,2.23 | 69.2,2.23 65.47,2.23 64.2,3.5 64.2,15.2 v65,16 | 69.2,4.6 69.2,2.23
  Bottom 0.5: v65,16 65,19.25 v63.75,20.5
AUDIO_BCK  (via drill 0.3)
  Top 0.2: U10.9 105.67,26.73 104.7,25.75 103.3,25.75 102.25,24.7 100.8,24.7 100.2,25.3 v97.6,25.3 | U1.38 93.5,26.75 v94.05,26.2
  Bottom 0.2: v94.05,26.2 96.7,26.2 v97.6,25.3
AUDIO_DATA
  Top 0.2: U10.7 104.62,27.38 104.85,27.15 104.85,26.5 104.5,26.15 103.1,26.15 102.05,25.1 101,25.1 100.4,25.7 98.55,25.7 95.5,28.75 U1.42
AUDIO_LRCK
  Top 0.2: U10.8 103.08,26.73 101.85,25.5 101.2,25.5 100.6,26.1 98.75,26.1 95.6,29.25 U1.43
BUS_A0
  Top 0.2: U1.41 94.3,28.25 96.4,26.15 96.4,19.6 93.35,16.55 92.75,16.55 92.62,16.43 U3.4
BUS_A0_5V
  Top 0.2: U3.20 91.97,6.58 90.6,5.2 90.6,3.52 J5.17
BUS_A1
  Top 0.2: U1.40 94.2,27.75 96,25.95 96,19.8 93.15,16.95 92.4,16.95 91.97,16.52 U3.5
BUS_A1_5V
  Top 0.2: U3.19 91.33,6.75 J5.16
BUS_A2
  Top 0.2: U1.39 94.1,27.25 95.6,25.75 95.6,20 92.95,17.35 91.9,17.35 91.33,16.77 U3.6
BUS_A2_5V
  Top 0.2: U3.18 90.67,8.03 88.05,5.4 88.05,3.53 J5.15
BUS_CS#
  Top 0.2: U1.28 87.75,24.85 86.9,24 85.45,24 84.8,23.35 84.8,17.4 | 84.8,17.4 88.05,17.4 88.72,16.73 U3.10 | U6.22 77.72,14.38 78.35,13.75 84.15,13.75 84.8,14.4 84.8,17.4
BUS_CS#_5V
  Top 0.2: J5.11 83,3.5 83,5.15 84.8,6.95 87.1,6.95 88.08,7.92 U3.14
BUS_D0
  Top 0.2: U1.27 87.25,24.95 86.7,24.4 85.25,24.4 84.8,23.95 83.85,23.95 82.35,22.45 82.35,16.9 82.92,16.32 U6.14
BUS_D0_5V
  Top 0.2: U6.10 82.28,8.57 81.7,8 81.7,4.8 J5.10
BUS_D1
  Top 0.2: U1.26 86.75,25.05 86.5,24.8 85.05,24.8 84.6,24.35 83.64,24.35 81.95,22.66 81.95,16.65 82.28,16.32 U6.15
BUS_D1_5V
  Top 0.2: J5.9 80.45,3.51 80.45,7.35 81.62,8.53 U6.9
BUS_D2
  Top 0.2: U1.25 85.2,25.55 84.4,24.75 83.45,24.75 81.55,22.85 81.55,15.47 U6.16
BUS_D2_5V
  Top 0.2: U6.8 80.97,8.47 79.2,6.7 J5.8
BUS_D3
  Top 0.2: U1.23 84.8,26.75 84.5,26.45 82.85,26.45 82.7,26.3 82.7,24.6 81.15,23.05 81.15,16.5 80.97,16.32 U6.17
BUS_D3_5V
  Top 0.2: U6.7 80.33,8.43 77.95,6.05 77.95,3.47 J5.7 79.19,2.06
BUS_D4
  Top 0.2: U1.21 84.8,27.75 84.5,28.05 80.7,28.05 80.1,27.45 80.1,25.05 80.75,24.4 80.75,16.75 80.33,16.32 U6.18
BUS_D4_5V
  Top 0.2: J5.6 76.65,5.35 79.67,8.38 U6.6
BUS_D5
  Top 0.2: U1.20 84.9,28.25 84.7,28.45 80.5,28.45 79.7,27.65 79.7,24.85 80.35,24.2 80.35,17 79.67,16.32 U6.19
BUS_D5_5V
  Top 0.2: J5.5 75.4,3.48 75.4,5.05 76.2,5.85 76.55,5.85 79.03,8.32 U6.5
BUS_D6
  Top 0.2: U1.19 85,28.75 84.9,28.85 80.3,28.85 79.3,27.85 79.3,24.65 79.95,24 79.95,17.25 79.03,16.32 U6.20
BUS_D6_5V
  Top 0.2: J5.4 74.42,4.77 75.9,6.25 76.35,6.25 78.38,8.28 U6.4
BUS_D7
  Top 0.2: U1.18 80.1,29.25 78.9,28.05 78.9,24.45 79.55,23.8 79.55,17.5 78.38,16.32 U6.21
BUS_D7_5V
  Top 0.2: J5.3 72.75,3.59 72.75,4.95 73.65,5.85 74.9,5.85 75.7,6.65 76.15,6.65 77.72,8.22 U6.3
BUS_IRQ#
  Top 0.2: U1.32 89.75,24.65 90.5,23.9 90.5,16.5 90.67,16.32 U3.7
BUS_IRQ#_5V
  Top 0.2: U3.17 90.03,8.07 86.81,4.86 J5.14
BUS_PHI2  (via drill 0.3)
  Top 0.2: U1.37 93,26.25 93.8,25.45 94.6,25.45 95.2,24.85 95.2,20.2 93,18 v92.65,18 | U3.2 93.92,16.52 94.55,17.15 v94.95,17.15 95.85,16.25 96.55,16.25 100,12.8 U12.2
  Bottom 0.2: v92.65,18 94.1,18 v94.95,17.15
BUS_PHI2_5V
  Top 0.2: R49.2 R50.2 93.82,6.7 J5.18
BUS_PHI2_5V_IN
  Top 0.2: R50.1 93.5,8.3 93.28,8.53 U3.22
BUS_RDY  (via drill 0.3)
  Top 0.2: U1.36 92.35,25.55 v92.95,24.95 | v94.55,23.85 94.8,23.6 94.8,20.4 93.05,18.65 92.25,18.65 v91.85,19.05 | v96.05,17 96.4,17 100.05,13.35 104.4,13.35 | 104.4,13.35 110.15,13.35 111,12.5 113.2,12.5 113.8,13.1 113.8,14.97 J9.3 | U3.3 93.28,14.53 93.55,14.25 95.05,14.25 95.55,14.75 v95.55,15.5 | U13.2 104.4,13.35
  Bottom 0.2: v92.95,24.95 94.05,23.85 v94.55,23.85 | v91.85,19.05 92.25,18.65 94.4,18.65 v96.05,17 96.05,16 v95.55,15.5
BUS_RDY_5V
  Top 0.2: R51.2 R52.2 100.35,4.25 96.45,4.25 J5.19
BUS_RDY_5V_OD
  Top 0.2: R52.1 101.55,8.3 100.75,7.5 93.7,7.5 92.62,8.57 U3.21
BUS_RES#_5V
  Top 0.2: U3.15 88.72,7.97 87.3,6.55 86.05,6.55 J5.12
BUS_RW#
  Top 0.2: U1.31 89.25,24.55 90.1,23.7 90.1,16.05 90.05,16 90.05,15.43 U3.8
BUS_RW#_5V  (via drill 0.3)
  Top 0.2: U9.2 71.35,9.95 71.8,10.4 v71.8,10.95 | v71.8,13.2 72.05,12.95 88.55,12.95 v88.75,13.15 | v88.75,10.95 89.3,10.95 89.38,10.88 U3.16 89.38,8.03 87.5,6.15 86.6,6.15 85.5,5.05 85.5,3.54 J5.13
  Bottom 0.2: v88.75,10.95 v88.75,13.15 | v71.8,10.95 v71.8,13.2
FLASH_SSEL_N
  Top 0.2: 51.35,14.63 U4.1 51.35,14.6 51.1,14.85 49,14.85 48.35,14.2 48.35,10.5 49.9,8.95 U11.8
FPGA_CDONE  (via drill 0.3)
  Top 0.2: U1.7 88.75,33.15 88.45,33.45 88.45,33.8 88.25,34 88.25,35.4 v88,35.65 | v84.5,35.65 83.6,35.65 R35.2 83.4,35.75 82.7,35.05 82.7,32.35 82.4,32.05 79.3,32.05 76.5,29.25 76.5,25.7 71.65,20.85 65.25,20.85 63.45,19.05 62.95,19.05 61.5,20.5 J3.2 59.6,18.95 v59.6,12.6 | U11.1 57.85,5.05 58,5.2 58,5.7 | 58,5.7 58.2,5.7 v59.15,6.65 | 58,5.7 U11.2 53.65,5.7 53,6.35 U11.12 | v58.35,10.1 59.15,9.3 v59.15,7.95
  Bottom 0.2: v88,35.65 v84.5,35.65 | v59.6,12.6 58.35,11.35 v58.35,10.1 | v59.15,7.95 v59.15,6.65
FPGA_CRESET_B  (via drill 0.3)
  Top 0.2: U1.8 88.25,33 88.05,33.2 88.05,33.6 87.5,34.15 v87.5,34.45 | R34.2 83.65,34.35 v84.5,34.35 84.5,33.55 82.6,31.65 79.5,31.65 76.9,29.05 76.9,25.5 75.6,24.2 v75.6,23.85 75.45,23.7 75.1,23.7 71.85,20.45 65.45,20.45 63.35,18.35 61.5,18.35 J3.3 | U3.9 89.38,16.68 88.25,17.8 86.6,17.8 v85.9,18.5 | v83.5,18.5 v83.5,20.35 | v78.5,22.65 v78.5,20.35
  Bottom 0.2: v87.5,34.45 87.4,34.35 v84.5,34.35 | v85.9,18.5 v83.5,18.5 | v83.5,20.35 v78.5,20.35 | v75.6,23.85 76.15,23.85 76.35,23.65 77.7,23.65 78.5,22.85 v78.5,22.65
GND  (via drill 0.3)
  Top 0.2: U3.12 87.4,15.43
  Top 0.3: U3.23 93.92,10.88 v93.95,10.9 | 87.4,15.43 v87.4,16.65 | U9.3 v70.7,8.5 | U10.4 104.92,29.32 v104.95,29.35 | U10.13 108.17,29.32 v108.05,29.45 | U11.7 v58,8.95 | U12.3 v98.65,12.1
  Top 0.5: C70.1 v68.55,13.3 | U8.2 v65.45,28.75 | C25.1 v61.8,27 61.8,26.3 R45.1 | C26.1 v72.85,29 | C7.1 v81.05,27.25 | C8.1 v81.05,25.65 | C13.1 v89.3,20.25 | C9.1 v91.3,20.25 | C10.1 v92.85,20.25 | C11.1 v94.45,35.95 C6.1 | C14.1 v87.8,20.25 | C23.1 v58.25,17.2 | U4.4 v52.4,10.8 | v86.75,31.25 v89,31.25 | v89,31.25 v91.25,31.25 v91.25,29 v91.25,26.75 v89,26.75 | v89,26.75 v86.75,26.75 | U1.49 v86.75,29 | U1.49 v89,31.25 | v89,26.75 U1.49 | U5.2 101.37,22.25 v102.45,22.25 | C5.1 v96,11.8 | C18.1 v101.3,17.45 | 67.9,6.7 67.8,6.8 C69.1 v67.6,5.7 | C19.1 v74.5,9.05 74.55,9 | C4.1 72.35,14.3 | U2.2 v66.7,9.5 | C17.1 v105.75,31.9 | C16.1 v107.25,31.9 | J7.3 14.65,34.25 v14.65,33.1 | C28.2 v17.15,28.9 | R24.2 v67,40.15 | R16.2 v67,34.65 | R23.1 v65.4,34.65 | v61.15,43.4 C2.1 62.15,43.35 62.15,41.55 | C1.1 62.15,41.55 | 62.15,41.55 v61.35,41.55 | C29.1 v53.25,3.35 | C24.1 v113.05,31.85 | C27.1 v113.05,28.65 | C30.1 v102.2,12.35 | C31.1 v106.6,12.35 | C21.1 v99.95,30.75 | C22.1 v99.95,27.85 | J6.5 104.8,57.58 v104.8,55.8
  Top 0.6: C12.1 v90.35,36.45 C15.1
  other vias: 72.3,14.3 77.45,13.65 85.25,13.65 79,10.95 90.05,14 97.5,13.5 90.2,10.95 83.5,17 77,16.85 80.7,35.9 84.1,31.9 87.5,43.5 91.5,43.5 85.5,9.5 112.5,47.5 28.35,29.15 7.5,2.5 2.5,7.5 7.5,12.5 2.5,17.5 7.5,22.5 12.5,17.5 12.5,7.5 17.5,2.5 17.5,12.5 17.5,22.5 27.5,22.5 37.5,22.5 42.5,17.5 32.5,17.5 22.5,17.5 27.5,12.5 37.5,12.5 42.5,7.5 32.5,7.5 22.5,7.5 27.5,2.5 37.5,2.5 47.5,2.5 2.5,37.5 2.5,47.5 7.5,52.5 17.5,52.5 17.5,42.5 12.5,37.5 12.5,47.5 7.5,42.5 12.5,57.5 22.5,57.5 27.5,52.5 22.5,47.5 27.5,42.5 22.5,37.5 12.5,27.5 17.5,27.5 32.5,47.5 37.5,42.5 32.5,37.5 37.5,32.5 27.5,32.5 47.5,32.5 57.5,32.5 42.5,37.5 52.5,27.5 57.5,2.5 47.5,22.5 52.5,37.5 47.5,42.5 42.5,47.5 47.5,52.5 42.5,57.5 32.5,57.5 52.5,57.5 62.5,57.5 57.5,52.5 62.5,47.5 57.5,42.5 57.5,22.5 67.5,52.5 72.5,57.5 82.5,57.5 92.5,57.5 102.5,57.5 97.5,52.5 77.5,52.5 102.5,47.5 102.5,37.5 107.5,52.5 107.5,47.5 112.5,57.5 107.5,2.5 97.5,2.5 107.5,22.5 112.5,27.5 97.5,30 28.35,27.85 28.35,26.55 54,42.5 55.8,42.5 46.1,46.05 51,41.15
  pour Bottom: 2,60 113,60 arc-90 115,58 115,2 arc-90 113,0 2,0 arc-90 0,2 0,58 arc-90
  pour Top: 2,60 113,60 arc-90 115,58 115,2 arc-90 113,0 2,0 arc-90 0,2 0,58 arc-90
N$1
  Top 0.2: R3.1B R1.1A
N$2
  Top 0.2: R3.2B R1.2A
N$3
  Top 0.2: R3.3B R1.3A
N$4
  Top 0.2: R3.4B R1.4A
N$5
  Top 0.2: R7.1B R2.1A
N$6
  Top 0.2: R7.2B R2.2A
N$7
  Top 0.2: U2.1 65.75,9.65 66.35,10.25 67.05,10.25 67.65,9.65 U2.3
  Top 0.5: C69.2 65.75,6.8 | 65.75,6.8 U2.1 | 65.75,6.8 65.9,6.65 R28.2
N$8
  Top 0.2: U6.2 77.08,8.62 76.8,8.35 73.35,8.35 72.9,8.8 U9.4
N$9
  Top 0.2: R30.1B R29.1A
N$10
  Top 0.2: R7.3B R2.3A
N$11
  Top 0.2: R7.4B R2.4A
N$12
  Top 0.35: R27.1 56.72,38.63 U7.6 59.62,38.63 60.25,38 60.25,34.85 R33.1
N$13
  Top 0.2: R3.2A R14.2B 70,33.4 69.6,33.4 69,32.8 68.6,32.8 R14.1A
N$14
  Top 0.2: U4.3 49.97,12.06 R43.2
N$15
  Top 0.3: R13.1 R45.2 63.4,26.3 63.4,27.8 U8.5
N$16
  Top 0.2: R3.3A R14.3B 70,34.2 69.6,34.2 69,33.6 68.6,33.6 R14.2A
N$17
  Top 0.2: R3.4A R14.4B 70,35 69.6,35 69,34.4 68.6,34.4 R14.3A
N$18
  Top 0.2: R7.1A R15.1B 70.1,36.05 69.85,35.8 68.75,35.8 68.5,35.55 R14.4A
N$19
  Top 0.3: U4.7 58.16,13.34 R44.2
N$20
  Top 0.5: U8.3 69.5,29.7 L1.1
N$21
  Top 0.2: R7.2A R15.2B 70,37.2 69.6,37.2 69,36.6 68.6,36.6 R15.1A
N$22
  Top 0.2: U8.1 65.3,27.8 64.7,28.4 64.7,28.85 63.85,29.7 U8.4
  Top 0.5: U8.4 C25.2 R37.2
N$23
  Top 0.35: U7.8 56.65,36.09 R32.1
N$24
  Top 0.35: C3.1 R33.2
N$25
  Top 0.2: R7.4A R15.4B 70,38.8 69.6,38.8 69,38.2 68.6,38.2 R15.3A
N$26
  Top 0.3: U10.3 101.67,29.98 C20.2
N$27
  Top 0.2: R30.2B R29.2A
N$28
  Top 0.2: R30.3B R29.3A
N$29
  Top 0.2: R15.2A 67.2,37.3 R16.1
N$30
  Top 0.2: R30.4B R29.4A
N$31
  Top 0.2: R30.1A R31.1B 70,40.2 69.6,40.2 69.35,39.95 69.35,39.35 69,39 68.6,39 R15.4A
N$32
  Top 0.2: R30.2A R31.2B 70,41 69.6,41 69,40.4 68.6,40.4 R31.1A
N$33
  Top 0.2: R30.3A R31.3B 70,41.8 69.6,41.8 69,41.2 68.6,41.2 R31.2A
N$34
  Top 0.2: R31.4A 67.1,42.7 R24.1
N$35
  Top 0.2: R30.4A R31.4B 70,42.6 69.6,42.6 69,42 68.6,42 R31.3A
N$36
  Top 0.35: U7.7 56.23,37.37 55,38.6 R26.1
N$37
  Top 0.5: R36.1 C2.2 63.9,41.65 C1.2 63.8,40.08 U7.4
N$38
  Top 0.3: R38.2 C17.2
  Top 0.5: C17.2 105.75,47.48 J6.4
N$39
  Top 0.3: R39.2 C16.2
  Top 0.5: J6.1 112.17,48.42 107.1,43.35 107.1,34.5 C16.2
N$40
  Top 0.3: U10.1 103.6,32.1 R38.1
N$41
  Top 0.3: U10.16 109.4,32.1 R39.1
N$42
  Top 0.3: U10.5 101.72,28.68 C20.1
N$43
  Top 0.2: R47.2 26.25,31.5 J7.8
N$44
  Top 0.2: R48.2 7.5,33.35 7.5,33.6 7.12,33.98 J7.9
N$45
  Top 0.3: U10.2 102.62,30.62 102.45,30.8 102.45,31.4 102.25,31.6 C21.2
N$46
  Top 0.2: U11.3 55.55,6.35 53.6,8.3 U11.9
N$47  (via drill 0.3)
  Top 0.2: U11.6 v55.15,8.3 | v53.85,7 53.2,7.65 U11.10 | U11.13 v52.7,5.7
  Bottom 0.2: v55.15,8.3 v53.85,7 52.7,5.85 v52.7,5.7
N$48
  Top 0.2: R49.1 99.35,8.95 U12.4
N$49
  Top 0.3: U10.14 110.97,29.98 C27.2
N$50
  Top 0.2: U13.4 103.75,8.95 R51.1
N$51
  Top 0.2: J7.2 12.1,34.23 12.1,30.65 16.85,25.9 42.2,25.9 49.85,18.25 50.35,18.25 R54.2
N$52
  Top 0.2: J7.5 19.6,34.23 19.6,30 22.4,27.2 45.3,27.2 50.7,21.8 R53.2
N$53
  Top 0.2: J7.1 9.62,34.02 11.7,31.95 11.7,30.45 16.65,25.5 42,25.5 47.55,19.95 R56.2
N$54
  Top 0.2: J7.7 R55.2
SD_SSEL_N
  Top 0.2: R40.2 R56.1 49.45,7.45 49.8,7.45 50.25,7 U11.11
SPI_MISO  (via drill 0.3)
  Top 0.2: 51.39,13.35 U4.2 53.34,13.34 54.5,14.5 54.5,18 | U1.17 80,29.75 78.5,28.25 78.5,23.9 v78.8,23.6 | R42.2 R55.1 24.55,28.95 25,28.5 46.25,28.5 54.5,20.25 54.5,18 | v76.65,24.3 76.5,24.15 76.5,23.8 75.9,23.2 75.2,23.2 72.05,20.05 65.65,20.05 61.5,15.9 J3.4 | 54.5,18 v57.35,18
  Bottom 0.2: v76.65,24.3 78.1,24.3 v78.8,23.6 | v57.35,18 59.27,18 J3.4
SPI_MOSI  (via drill 0.3)
  Top 0.2: U4.5 | U1.14 79.7,31.25 77.3,28.85 77.3,24 76.1,22.8 75.4,22.8 72.25,19.65 65.85,19.65 62.8,16.6 62.8,14.55 61.5,13.25 J3.5 | U4.5 57,10.79 57,10.8 59,10.8 v59.7,10.1 | R54.1 R41.2 53.3,15.3 v53.3,14.7 | v53.75,12.7 55.65,10.8 U4.5
  Bottom 0.2: v53.3,14.7 53.3,13.15 v53.75,12.7 | v59.7,10.1 59.7,10.95 61.5,12.75 J3.5
SPI_SCK  (via drill 0.3)
  Top 0.2: 56.56,12 U4.6 | U1.15 79.8,30.75 77.7,28.65 77.7,23.8 76.3,22.4 75.6,22.4 72.45,19.25 66.05,19.25 63.2,16.4 63.2,14.35 62.8,13.95 62.8,12 J3.6 60.11,10.69 58.7,12.1 56.66,12.1 U4.6 | 56.64,12.05 U4.6 | U4.6 56.27,12.06 55,13.33 v55,14 | R53.1 53.65,18.15 v53.65,16.2
  Bottom 0.2: v53.65,16.2 55,14.85 v55,14
SPI_SSEL_N
  Top 0.2: U1.16 79.9,30.25 78.1,28.45 78.1,23.6 76.5,22 75.8,22 72.65,18.85 69.65,18.85 | U11.4 57.85,7 58,7.15 58,7.3 | 58,7.3 58,7.5 57.85,7.65 U11.5 | 69.65,18.85 66.25,18.85 63.6,16.2 63.6,14.1 63.2,13.7 63.2,11.7 62.8,11.3 62.8,9.45 J3.7 61.4,8.15 60.55,7.3 58,7.3 | R46.2 69.65,18.85
SYSCLK  (via drill 0.3)
  Top 0.2: U1.35 91.25,25.1 92.2,24.15 93.65,24.15 v94.3,24.8 | v97.8,22.25 99.13,22.25 U5.3 99.15,23.5 99.55,23.9 104.9,23.9 106.5,25.5 110.5,25.5 111,26 111,27 110.62,27.38 U10.10
  Bottom 0.2: v97.8,22.25 95.25,24.8 v94.3,24.8
UART_RX  (via drill 0.3)
  Top 0.2: U1.34 90.75,25 92,23.75 93.65,23.75 94.4,23 94.4,20.6 93.3,19.5 93.1,19.5 92.9,19.3 v92.75,19.3 | v96,18 100.25,13.75 112.48,13.75 J9.2
  Bottom 0.2: v92.75,19.3 94.7,19.3 v96,18
VGA_B
  Top 0.5: R22.2 R21.2 R20.2 R19.2 93.25,41.55 92.15,42.65 89.9,42.65 88.2,44.35 84.44,44.35 J1.3
VGA_B0  (via drill 0.3)
  Top 0.2: U1.46 93.1,30.75 94.6,32.25 95.95,32.25 96.9,33.2 96.9,37.55 v97.85,38.5 R22.1 | R29.4B v77.65,42.7
  Bottom 0.2: v97.85,38.5 93.6,42.75 77.7,42.75 v77.65,42.7
VGA_B1  (via drill 0.3)
  Top 0.2: U1.47 93,31.25 94.4,32.65 95.75,32.65 96.5,33.4 96.5,38.35 v96.35,38.5 R21.1 | R29.3B v77.1,41.9
  Bottom 0.2: v96.35,38.5 92.5,42.35 79,42.35 78.55,41.9 v77.1,41.9
VGA_B2  (via drill 0.3)
  Top 0.2: U1.48 92.9,31.75 94.2,33.05 95.55,33.05 96.1,33.6 96.1,37.25 v94.85,38.5 R20.1 | R29.2B v77.65,41.1
  Bottom 0.2: v94.85,38.5 91.4,41.95 79.2,41.95 78.35,41.1 v77.65,41.1
VGA_B3  (via drill 0.3)
  Top 0.2: U1.2 91.25,32.9 91.6,33.25 92.25,33.25 92.8,33.8 92.8,38.05 v93.25,38.5 R19.1 | R29.1B v77.1,40.3
  Bottom 0.2: v93.25,38.5 90.2,41.55 79.4,41.55 78.15,40.3 v77.1,40.3
VGA_G
  Top 0.5: R18.2 R17.2 R12.2 R11.2 86.85,42 86.05,42.8 83.7,42.8 J1.2
VGA_G0  (via drill 0.3)
  Top 0.2: U1.3 90.75,33 91.4,33.65 92.05,33.65 92.4,34 92.4,37.75 v91.65,38.5 R18.1 | R2.4B v77.65,38.9
  Bottom 0.2: v91.65,38.5 89,41.15 80.7,41.15 78.45,38.9 v77.65,38.9
VGA_G1  (via drill 0.3)
  Top 0.2: U1.4 90.25,33.1 91.2,34.05 91.85,34.05 92,34.2 92,37.25 91.8,37.45 91.1,37.45 v90.05,38.5 R17.1 | R2.3B v77.1,38.1
  Bottom 0.2: v90.05,38.5 87.8,40.75 80.9,40.75 78.25,38.1 v77.1,38.1
VGA_G2  (via drill 0.3)
  Top 0.2: U1.6 89.25,33.25 88.85,33.65 88.85,34 88.65,34.2 88.65,38.3 v88.45,38.5 R12.1 | R2.2B v77.65,37.3
  Bottom 0.2: v88.45,38.5 86.6,40.35 81.1,40.35 78.45,37.7 78.05,37.7 v77.65,37.3
VGA_G3  (via drill 0.3)
  Top 0.2: U1.9 87.75,32.9 87.65,33 87.65,33.35 86.85,34.15 v86.85,38.5 R11.1 | R2.1B v77.1,36.5
  Bottom 0.2: v86.85,38.5 85.4,39.95 81.3,39.95 77.85,36.5 v77.1,36.5
VGA_HS
  Top 0.3: R5.2 99.45,37.55 100,38.1 100,42.45 98.9,43.55 95.55,43.55 90.75,48.35 90.75,52 89.1,53.65 85.31,53.65 J1.13
VGA_HSYNC
  Top 0.2: U1.44 92.5,29.8 93.35,29.8 95,31.45 96.35,31.45 98.4,33.5 98.6,33.5 R5.1
VGA_R
  Top 0.5: R10.2 R9.2 R8.2 R4.2 80.45,43.77 J1.1
VGA_R0  (via drill 0.3)
  Top 0.2: U1.10 87.25,33.15 86.45,33.95 86.45,37.3 v85.25,38.5 R10.1 | R1.4B v77.65,35.1
  Bottom 0.2: v85.25,38.5 84.2,39.55 81.5,39.55 77.65,35.7 v77.65,35.1
VGA_R1  (via drill 0.3)
  Top 0.2: U1.11 86.75,33.05 86.05,33.75 86.05,36.25 84.5,37.8 84.3,37.8 83.65,38.45 v83.65,38.5 R9.1 | R1.3B v77.1,34.3
  Bottom 0.2: v83.65,38.5 83,39.15 81.7,39.15 78.35,35.8 78.35,34.85 77.8,34.3 v77.1,34.3
VGA_R2  (via drill 0.3)
  Top 0.2: U1.12 86.25,32.95 85.65,33.55 85.65,36.05 84.3,37.4 83.15,37.4 v82.05,38.5 R8.1 | R1.2B v77.65,33.5
  Bottom 0.2: v77.65,33.5 78.75,34.6 78.75,35.6 81.65,38.5 v82.05,38.5 81.7,38.5
VGA_R3
  Top 0.2: 80.45,39.7 R4.1 80.45,37 | U1.13 85.25,31.75 85.25,35.85 84.1,37 80.45,37 | R1.1B 77.8,32.7 78.3,33.2 78.3,34.85 80.45,37
VGA_VS
  Top 0.3: J1.14 86.69,52.75 88.4,52.75 89.75,51.4 89.75,47.9 95,42.65 98.5,42.65 99.1,42.05 99.1,38.55 97.85,37.3 R6.2
VGA_VSYNC
  Top 0.2: U1.45 93.2,30.25 94.8,31.85 96.15,31.85 97.85,33.55 R6.1
VIDEO_C
  Top 0.35: R27.2 56.6,46.7 J4.4
VIDEO_CHROMA  (via drill 0.3)
  Top 0.2: R15.3B v70.9,38.1 R7.3A | v67.3,38.7 R25.2 65.31,38.62 63.65,38.62 U7.3
  Bottom 0.2: v70.9,38.1 67.9,38.1 v67.3,38.7
VIDEO_COMP
  Top 0.35: C3.2 R32.2 38.55,52.5 J2.S
VIDEO_LUMA
  Top 0.2: R3.1A R14.1B 69.9,32.7 69.25,32.05 67.8,32.05 65.9,33.95 63.95,33.95 62.4,35.5 62.4,36.1 | R23.2 65.14,37.37 U7.2 62.66,37.37 62.4,37.1 62.4,36.1 | U7.1 62.41,36.09 62.4,36.1
VIDEO_Y
  Top 0.35: R26.2 55,46.1 J4.3

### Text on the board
tPlace: 1 | VERA module | rev1 | by Frank van den Hoef (C) 2019 | 1
bPlace: GND | D6 | D4 | D2 | D0 | RES# | IRQ# | A1 | PHI2 | GND | 5V | D7 | D5 | D3 | D1 | CS# | RW# | A2 | A0 | RDY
